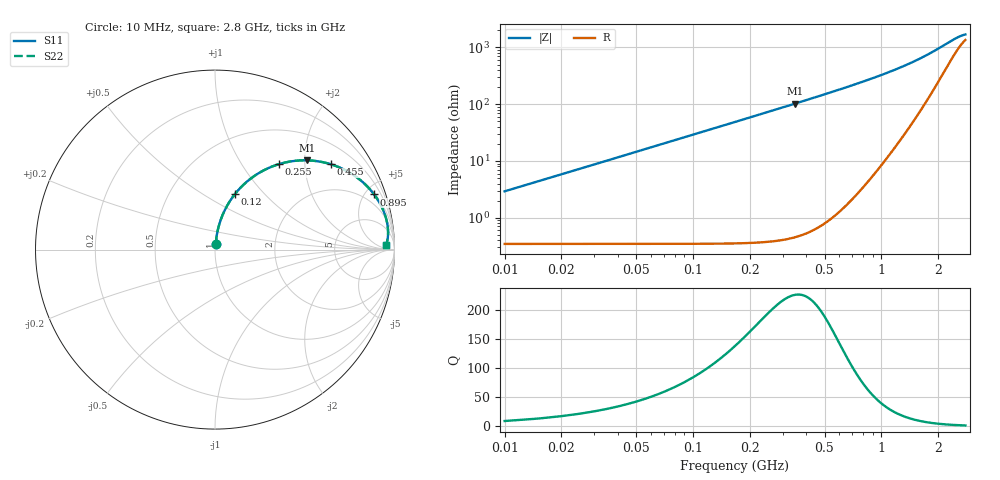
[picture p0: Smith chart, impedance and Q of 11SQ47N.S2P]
! Coilcraft 1111SQ-47N Air Core Inductor
! 15 MAR 2012
# MHZ S MA R 50
!Freq  MagS11  AngS11  MagS21  AngS21  MagS12  AngS12  MagS22  AngS22
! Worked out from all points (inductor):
!   559 points, 10 MHz to 2.8 GHz, reference 50 ohm
!   read as one part in series: L = 46.1 nH near 20 MHz
!   highest Q = 226 at 350 MHz (marker M1), where L = 46.8 nH
!   S11 on the Smith chart (normalised r, x): 10 MHz: 1.01, +0.06; 120 MHz: 1.01, +0.70; 255 MHz: 1.01, +1.49; 455 MHz: 1.02, +2.70; 895 MHz: 1.12, +5.72; 2.8 GHz: 31, +19
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10  0.02904 81.6  0.9961 -1.7  0.9961 -1.7  0.02904 81.6
15  0.04337 83.0  0.9956 -2.5  0.9956 -2.5  0.04337 83.0
25  0.07202 83.1  0.994 -4.1  0.994 -4.1  0.07202 83.1
30  0.0863 82.8  0.9928 -5.0  0.9928 -5.0  0.0863 82.8
40  0.1147 81.7  0.99 -6.6  0.99 -6.6  0.1147 81.7
50  0.1429 80.4  0.9863 -8.2  0.9863 -8.2  0.1429 80.4
65  0.1844 78.3  0.9795 -10.6  0.9795 -10.6  0.1844 78.3
80  0.2251 76.1  0.971 -13.0  0.971 -13.0  0.2251 76.1
120  0.3276 70.3  0.9415 -19.1  0.9415 -19.1  0.3276 70.3
180  0.4622 62.1  0.8836 -27.5  0.8836 -27.5  0.4622 62.1
255  0.5954 53.1  0.8004 -36.6  0.8004 -36.6  0.5954 53.1
350  0.7152 44.1  0.6958 -45.7  0.6958 -45.7  0.7152 44.1
455  0.8016 36.4  0.594 -53.3  0.594 -53.3  0.8016 36.4
475  0.8141 35.2  0.5766 -54.5  0.5766 -54.5  0.8141 35.2
660  0.8924 26.3  0.4437 -63.2  0.4437 -63.2  0.8924 26.3
895  0.9382 19.1  0.3293 -69.8  0.3293 -69.8  0.9382 19.1
940  0.9434 18.1  0.3121 -70.7  0.3121 -70.7  0.9434 18.1
1405  0.9684 10.6  0.1875 -75.1  0.1875 -75.1  0.9684 10.6
1870  0.9701 6.4  0.1167 -72.1  0.1167 -72.1  0.9701 6.4
2335  0.9638 3.6  0.07496 -59.5  0.07496 -59.5  0.9638 3.6
2585  0.959 2.5  0.06218 -47.6  0.06218 -47.6  0.959 2.5
2800  0.9544 1.7  0.05636 -35.3  0.05636 -35.3  0.9544 1.7
